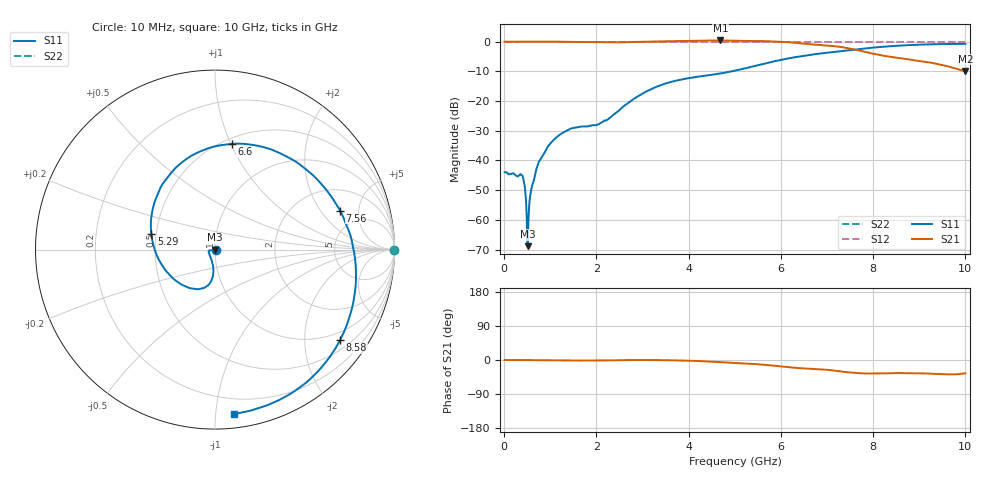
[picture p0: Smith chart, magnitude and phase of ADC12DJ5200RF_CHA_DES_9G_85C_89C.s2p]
! Texas Instruments, Inc.
! ADC12DJ5200RF - CH A S-Parameters (DES Mode, Fs = 9 GSPS, 85 degC case, 89 degC juntion)
! Port 1 represents the 100-ohm differenal input, Port 2 the digital output
! freq  dbS11  angS11  dbS21 angS21 dbS12 angS12 dbS22 angS22
# HZ S DB R 100
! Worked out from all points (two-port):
!   1000 points, 10 MHz to 10 GHz, reference 100 ohm
!   highest |S21| = 0.42 dB at 4.69 GHz (marker M1); lowest = -9.9 dB at 10 GHz (marker M2)
!   |S21| within 3 dB of the highest: start of sweep to 7.583 GHz
!   lowest |S11| = -68.9 dB at 510 MHz (marker M3), VSWR 1.00, Z = 100 - j0.0713 ohm
!   |S11| at or under -10 dB: start of sweep to 4.932 GHz
!   |S22| runs from 0.0 to 0.0 dB; largest |S21 - S12| = 0.76
!   S11 on the Smith chart (normalised r, x): 10 MHz: 1.01, -0.00; 5.29 GHz: 0.47, +0.10; 6.6 GHz: 0.55, +1.01; 7.56 GHz: 3.35, +3.13; 8.58 GHz: 0.75, -2.91; 10 GHz: 0.09, -1.12
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1e7  -43.98 -7.6  0.00 0.0  0.00 0.0  0.00 0.0
3.8e8  -44.92 -10.5  0.03 -0.2  0.00 0.0  0.00 0.0
4.3e8  -47.24 -0.5  0.03 -0.2  0.00 0.0  0.00 0.0
4.7e8  -52.81 6.8  0.03 -0.3  0.00 0.0  0.00 0.0
5.1e8  -68.87 -81.6  0.04 -0.3  0.00 0.0  0.00 0.0
6e8  -48.82 -136.8  0.05 -0.4  0.00 0.0  0.00 0.0
7.1e8  -42.37 -157.4  0.04 -0.4  0.00 0.0  0.00 0.0
9.4e8  -35.52 -169.1  0.07 -0.8  0.00 0.0  0.00 0.0
1.26e9  -30.80 -171.7  0.01 -1.4  0.00 0.0  0.00 0.0
1.68e9  -28.56 -163.4  -0.11 -1.4  0.00 0.0  0.00 0.0
2.24e9  -26.25 -119.8  -0.17 -1.2  0.00 0.0  0.00 0.0
3.34e9  -14.98 -96.9  0.10 -0.3  0.00 0.0  0.00 0.0
4.69e9  -10.70 -152.5  0.42 -5.7  0.00 0.0  0.00 0.0
5.01e9  -9.74 -174.4  0.34 -8.0  0.00 0.0  0.00 0.0
5.29e9  -8.74 165.9  0.24 -9.6  0.00 0.0  0.00 0.0
5.9e9  -6.49 126.2  0.04 -15.6  0.00 0.0  0.00 0.0
6.6e9  -4.49 81.1  -0.77 -23.0  0.00 0.0  0.00 0.0
6.67e9  -4.33 76.5  -0.90 -23.5  0.00 0.0  0.00 0.0
7.56e9  -2.73 17.4  -2.51 -33.6  0.00 0.0  0.00 0.0
8.34e9  -1.56 -25.8  -5.02 -35.0  0.00 0.0  0.00 0.0
8.58e9  -1.31 -35.9  -5.49 -34.6  0.00 0.0  0.00 0.0
1e10  -0.71 -83.2  -9.85 -35.3  0.00 0.0  0.00 0.0
